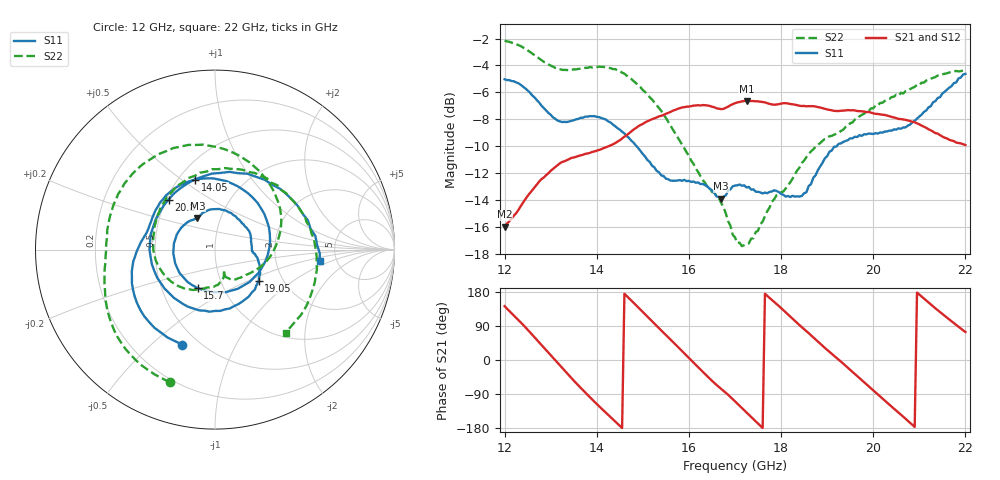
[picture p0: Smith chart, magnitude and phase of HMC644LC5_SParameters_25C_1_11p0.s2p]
!Analog Devices Inc..
!GaAs MMIC 5-BIT DIGITAL PHASE SHIFTER, 15 -8.5 GHz
!Filename: HMC644LC5_sparm_25C_1_0.s2p
!  :25C = 25degC
!  :_1_ = Sn1
!  :_11p0  = 11.25deg
!Device type:
!2 Port Calibration to sma connectors
!Phase Shifter:  0.000
!	TA = +25deg C, 50 Ohm System, Control Voltage = 0/-3V
!Freq	S11	S11	S21	S21	S12	S12	S22	S22
! GHz	Mag dB	Degrees	Mag dB	Degrees	Mag dB	Degrees	Mag dB	Degrees
# GHZ S DB R 50.0
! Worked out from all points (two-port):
!   201 points, 12 GHz to 22 GHz, reference 50 ohm
!   highest |S21| = -6.64 dB at 17.25 GHz (marker M1); lowest = -16.0 dB at 12 GHz (marker M2)
!   |S21| within 3 dB of the highest: 14.46 GHz to 21.75 GHz (7.29 GHz wide, 40.3 % of centre)
!   lowest |S11| = -13.9 dB at 16.7 GHz (marker M3), VSWR 1.50, Z = 38.8 + j14.2 ohm
!   |S11| at or under -10 dB: 14.86 GHz to 19.21 GHz (4.349 GHz wide, 25.5 % of centre)
!   |S22| runs from -17.4 to -2.1 dB; largest |S21 - S12| = 0.003
!   S11 on the Smith chart (normalised r, x): 12 GHz: 0.41, -0.63; 14.05 GHz: 0.60, +0.56; 15.7 GHz: 0.76, -0.34; 19.05 GHz: 1.51, -0.59; 20.8 GHz: 0.51, +0.33; 22 GHz: 3.68, -0.74
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12  -5.03 -109.0  -16.00 142.0  -15.99 142.1  -2.14 -108.8
12.45  -5.71 -149.8  -13.95 86.6  -13.95 86.7  -2.75 -138.6
13.1  -7.97 168.9  -11.55 -0.7  -11.55 -0.7  -4.18 -172.1
13.7  -7.89 135.5  -10.65 -79.6  -10.64 -79.6  -4.22 158.9
14.05  -7.85 105.6  -10.29 -122.0  -10.30 -121.9  -4.09 137.2
14.7  -9.40 35.7  -9.05 163.1  -9.02 163.2  -4.88 88.3
15.35  -11.95 -59.6  -7.79 84.0  -7.80 84.1  -7.16 36.0
15.7  -12.58 -114.5  -7.31 42.0  -7.29 42.2  -9.04 8.0
16.15  -12.73 178.1  -6.98 -12.9  -6.98 -12.8  -11.67 -24.1
16.7  -13.92 119.1  -7.25 -76.3  -7.23 -76.1  -14.23 -57.8
17  -12.94 94.5  -6.81 -109.0  -6.80 -108.9  -16.79 -69.8
17.25  -13.08 70.1  -6.64 -138.6  -6.64 -138.6  -17.28 -67.8
17.85  -13.29 28.2  -6.92 153.3  -6.88 153.1  -13.96 -88.7
18.3  -13.76 3.6  -6.92 103.0  -6.90 103.0  -12.11 -115.7
18.7  -12.35 -11.1  -7.03 59.7  -7.04 59.6  -10.24 -147.8
19.05  -10.42 -36.0  -7.31 21.4  -7.28 21.5  -9.27 -179.8
19.45  -9.56 -71.7  -7.32 -20.4  -7.35 -20.2  -8.52 146.2
19.8  -9.12 -104.6  -7.43 -58.5  -7.42 -58.5  -7.60 114.2
20.35  -8.85 -166.7  -7.78 -118.0  -7.77 -117.8  -6.50 65.7
20.8  -8.40 132.9  -8.14 -165.8  -8.12 -165.8  -5.76 30.7
21.3  -6.74 66.7  -8.93 141.4  -8.91 141.5  -4.92 -4.0
22  -4.63 -6.4  -9.92 74.0  -9.93 73.7  -4.32 -49.8
